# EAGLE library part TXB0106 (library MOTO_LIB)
6-BIT BIDIRECTIONAL VOLTAGE-LEVEL TRANSLATOR FOR PUSH-PULL APPLICATIONS
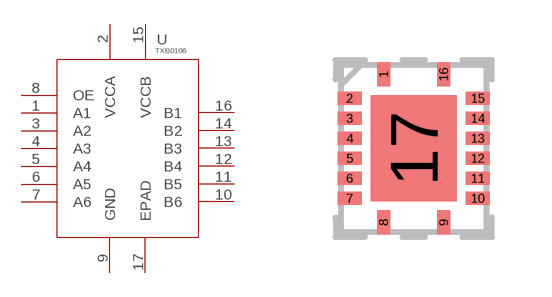
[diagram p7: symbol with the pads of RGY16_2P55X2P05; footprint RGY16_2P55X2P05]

Designator prefix U

## TXB0106 (MPN: TXB0106RGYR; SUPPLIER: TEXAS INSTRUMENTS)  [RGY16_2P55X2P05]
1  A1
2  VCCA  pwr
3  A2
4  A3
5  A4
6  A5
7  A6
8  OE  in
9  GND  pwr
10  B6
11  B5
12  B4
13  B3
14  B2
15  VCCB  pwr
16  B1
17  EPAD  pas

## Footprint RGY16_2P55X2P05 (pad centres in mm)
smd 0.33 x 0.6: 1 -0.75,1.85; 8 -0.75,-1.85; 9 0.75,-1.85; 16 0.75,1.85
smd 0.6 x 0.33: 2 -1.6,1.25; 3 -1.6,0.75; 4 -1.6,0.25; 5 -1.6,-0.25; 6 -1.6,-0.75; 7 -1.6,-1.25; 10 1.6,-1.25; 11 1.6,-0.75; 12 1.6,-0.25; 13 1.6,0.25; 14 1.6,0.75; 15 1.6,1.25
smd 2.15 x 2.65: 17 0,0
